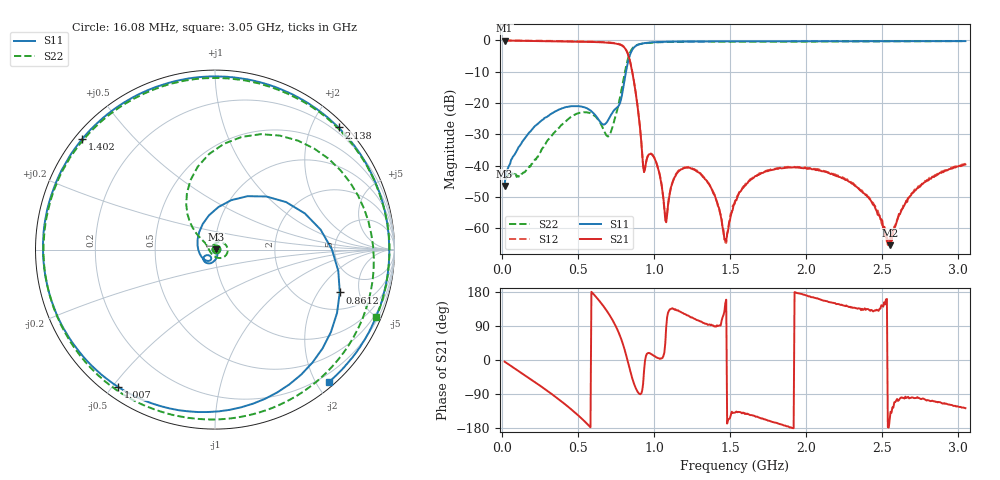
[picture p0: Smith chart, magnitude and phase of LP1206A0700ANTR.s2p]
# MHz S dB R 50
!  Frq	S11(dB)	S11(deg)	S21(dB)	S21(deg)	S12(dB)	S12(deg)	S22(dB)	S22(deg)
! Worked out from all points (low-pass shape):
!   500 points, 16.08 MHz to 3.05 GHz, reference 50 ohm
!   highest |S21| = -0.05 dB at 16.08 MHz (marker M1); lowest = -65.5 dB at 2.551 GHz (marker M2)
!   |S21| within 3 dB of the highest: start of sweep to 815.3 MHz
!   lowest |S11| = -46.5 dB at 16.08 MHz (marker M3), VSWR 1.01, Z = 50.4 + j0.161 ohm
!   |S11| at or under -10 dB: start of sweep to 815.4 MHz
!   |S22| runs from -44.5 to -0.2 dB; largest |S21 - S12| = 0.013
!   S11 on the Smith chart (normalised r, x): 16.08 MHz: 1.01, +0.00; 861.2 MHz: 3.06, -3.19; 1.007 GHz: 0.04, -0.52; 1.402 GHz: 0.02, +0.36; 2.138 GHz: 0.11, +2.43; 3.05 GHz: 0.08, -2.17
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16.08  -46.51 19.8  -0.05 -4.5  -0.03 -4.4  -44.55 10.5
301.84  -24.18 -92.8  -0.24 -82.7  -0.16 -82.7  -31.76 115.0
526.8  -21.20 -136.5  -0.43 -155.8  -0.32 -155.7  -22.96 0.8
642.32  -25.83 -143.2  -0.59 154.8  -0.48 154.9  -26.13 -69.0
739.6  -22.20 -127.6  -0.97 95.8  -0.84 95.8  -25.51 151.7
806.48  -12.48 85.5  -2.41 27.0  -2.27 27.0  -10.52 122.6
861.2  -2.67 -19.0  -11.34 -54.4  -11.19 -54.4  -2.35 52.7
934.16  -0.90 -88.7  -42.10 -28.6  -41.99 -29.6  -0.96 -11.2
1007.12  -0.57 -125.2  -38.17 9.6  -37.99 8.7  -0.67 -49.8
1031.44  -0.52 -134.5  -41.79 4.6  -41.75 3.3  -0.60 -60.3
1080.08  -0.45 -150.5  -58.12 87.0  -57.02 82.1  -0.52 -79.0
1201.68  -0.36 178.2  -40.69 121.3  -40.58 120.6  -0.41 -117.0
1402.32  -0.33 140.1  -49.88 88.7  -49.80 90.5  -0.40 -164.6
1469.2  -0.33 129.4  -63.61 149.8  -64.56 138.7  -0.39 -178.0
1536.08  -0.33 119.4  -51.10 -138.2  -50.81 -136.8  -0.39 169.5
2040.72  -0.30 55.5  -41.20 165.7  -40.84 165.4  -0.39 92.8
2138  -0.28 44.7  -42.12 155.3  -42.05 154.8  -0.38 80.2
2417.68  -0.26 14.8  -50.63 131.5  -50.48 133.8  -0.33 46.6
2545.36  -0.26 1.6  -65.02 -178.4  -65.75 -172.8  -0.30 32.1
2551.44  -0.25 1.0  -65.48 -156.1  -63.71 -154.1  -0.31 31.4
2727.76  -0.24 -17.0  -47.53 -100.1  -47.42 -100.3  -0.27 11.9
3050  -0.24 -49.4  -39.66 -127.1  -39.42 -127.4  -0.23 -22.7
